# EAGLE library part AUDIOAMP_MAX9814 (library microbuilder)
MAX9814 - Mono Microphone Amplifier with AGC
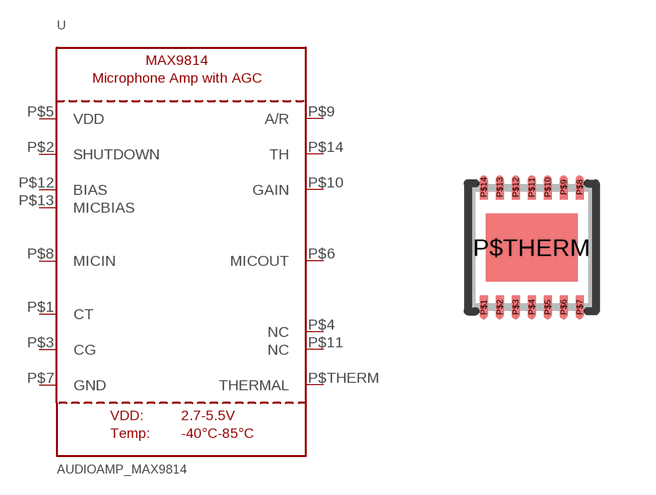
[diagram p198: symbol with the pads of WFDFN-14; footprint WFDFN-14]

Designator prefix U

## AUDIOAMP_MAX9814  [WFDFN-14]
P$1  CT
P$2  SHUTDOWN
P$3  CG
P$4  NC
P$5  VDD
P$6  MICOUT
P$7  GND
P$8  MICIN
P$9  A/R
P$10  GAIN
P$11  NC
P$12  BIAS
P$13  MICBIAS
P$14  TH
P$THERM  THERMAL

## Footprint WFDFN-14 (pad centres in mm)
14-WFDFN 3x3mm 0.4mm Pitch Source: http://datasheets.maxim-ic.com/en/ds/MAX9814.pdf
smd 0.2 x 0.6: P$1 -1.2,-1.5; P$2 -0.8,-1.5; P$3 -0.4,-1.5; P$4 0,-1.5; P$5 0.4,-1.5; P$6 0.8,-1.5; P$7 1.2,-1.5; P$8 1.2,1.5; P$9 0.8,1.5; P$10 0.4,1.5; P$11 0,1.5; P$12 -0.4,1.5; P$13 -0.8,1.5; P$14 -1.2,1.5
smd 2.3 x 1.7: P$THERM 0,0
